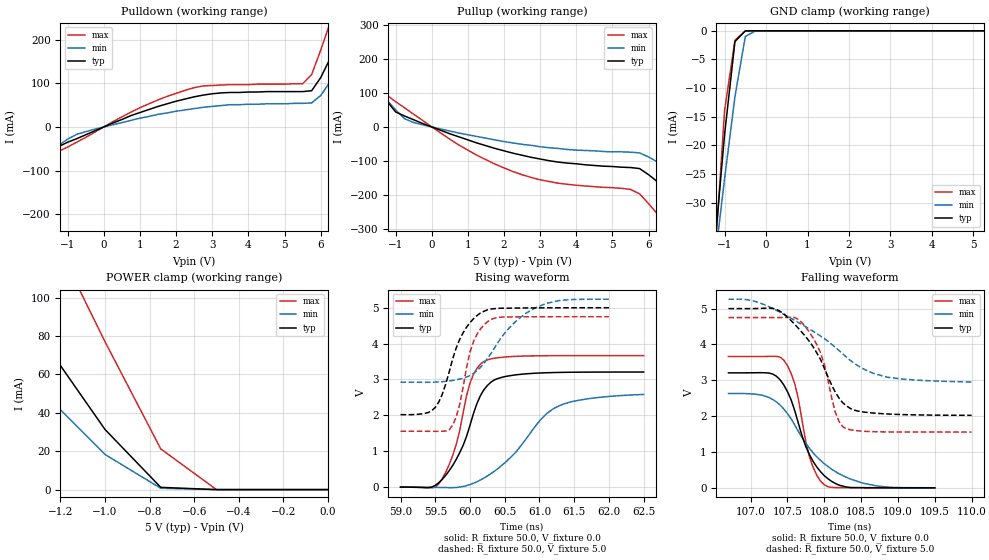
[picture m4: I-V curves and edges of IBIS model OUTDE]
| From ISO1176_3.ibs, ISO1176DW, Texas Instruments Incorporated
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[Model]   OUTDE
Model_type   3-state
| Signals   ISODE
Vmeas = 2.2V   |Reference voltage for timing measurements
Cref = 15pF   |Timing specification test load capacitance value
Vref = 0   |Timing specification test load voltage; GND
| variable   typ   min   max
C_comp   2.1pF   1.7pF   2.5pF
|   typ   min   max
[Temperature Range]   25.0   -40   125
[Voltage range]   5.0V   5.25V   4.75V
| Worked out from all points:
|   slope of the pulldown table from 0 to 0.75 V, typ, clamps not added: 28.8 ohm
|   slope of the pullup table from 0 to 0.75 V, typ, clamps not added: 25.9 ohm
|   GND clamp passes 1 mA (typ) near -0.63 V on its own axis
|   POWER clamp passes 1 mA (typ) near -0.71 V on its own axis
|   rising waveform, R_fixture 50.0, V_fixture 0.0: 20-80 % time 393ps typ, 714ps min, 285ps max; typ from 0.001 V to 3.21 V
|   falling waveform, R_fixture 50.0, V_fixture 0.0: 20-80 % time 354ps typ, 607ps min, 227ps max; typ from 3.21 V to 0 V
|   rising waveform, R_fixture 50.0, V_fixture 5.0: 20-80 % time 327ps typ, 586ps min, 227ps max; typ from 2.02 V to 5 V
|   falling waveform, R_fixture 50.0, V_fixture 5.0: 20-80 % time 497ps typ, 961ps min, 272ps max; typ from 5 V to 2.02 V
[Pulldown]
|   Voltage   I(typ)  I(min)  I(max)
-5.25V    -390mA     -298mA     -529mA
-4.25V    -301mA     -233mA     -406mA
-3.5V     -235mA     -185mA     -315mA
-2.75V    -169mA     -137mA     -223mA
-1.5V     -63mA      -58mA      -75mA
-750mV    -27mA      -17mA      -35mA
2.5V      69mA       42mA       90mA
5.5V      81mA       54mA       99mA
6.25V     155mA      102mA      236mA
6.75V     243mA      165mA      358mA
7.25V     333mA      231mA      483mA
10.5V     958mA      685mA      1.342A
[Pullup]
|   Voltage   I(typ)  I(min)  I(max)
| Note that the[Pullup]voltage table is referenced to Vcc
| and is calculated using Vtable=Vcc - Vmeasured.
-5.25V    791mA      609mA      1.061A
-3V       385mA      309mA      505mA
-2.5V     295mA      242mA      382mA
-2.25V    250mA      209mA      321mA
-1.25V    77mA       80mA       94mA
-1V       44mA       50mA       74mA
2.25V     -77mA      -47mA      -131mA
5.75V     -122mA     -76mA      -196mA
6.5V      -184mA     -119mA     -287mA
7.75V     -297mA     -201mA     -444mA
9.25V     -435mA     -301mA     -634mA
10.5V     -549mA     -384mA     -793mA
[GND_clamp]
|   Voltage   I(typ)   I(min)   I(max)
| Outputs in High Impedance (off)
-5.25V    -389mA     -298mA     -529mA
-1.25V    -38.6mA    -41.1mA    -41.5mA
-1V       -18.1mA    -25.8mA    -13.9mA
-750mV    -1.88mA    -11.5mA    -1.64mA
-500mV    -9.27uA    -986uA     -29.5uA
-250mV    -2.83nA    -1.59uA    -2.12nA
5.25V     59.6pA     2.04nA     374pA
[POWER_clamp]
|   Voltage  I(typ)   I(min)   I(max)
| Note that the [POWER_clamp] voltage table is referenced to Vcc
| and is calculated using Vtable = Vcc - Vmeasured.
| Outputs in Tri-state.
-5.25V    791mA      575mA      1.12A
-1.75V    160mA      111mA      258mA
-1.5V     116mA      78.7mA     197mA
-1.25V    72.9mA     47.4mA     136mA
-1V       31.3mA     18.3mA     77mA
-750mV    1.18mA     693uA      21.2mA
-500mV    96.1nA     841nA      9.4uA
0V        47.1pA     1.11nA     46.9pA
[Ramp]
|   typ   min   max
dV/dt_r   1.94V/0.39ns   1.59V/0.73ns   2.22V/0.28ns
dV/dt_f   1.94V/0.35ns   1.59V/0.61ns   2.22V/0.23ns
R_load = 50
[Rising Waveform]
R_fixture = 50.0
V_fixture = 0.0
C_fixture = 0p
L_fixture = 0n
|   V(typ)   V(min)   V(max)
59ns      627.5uV    504.9uV    -196.9nV
59.45ns   2.406mV    -5.873mV   -21.29mV
59.6ns    214.8mV    -10.74mV   231.2mV
59.8ns    766.5mV    -10.7mV    1.179V
60ns      1.726V     70.81mV    2.901V
60.2ns    2.712V     250.9mV    3.501V
60.45ns   3.055V     593.2mV    3.616V
61.2ns    3.193V     2.185V     3.663V
61.6ns    3.204V     2.433V     3.664V
62.5ns    3.208V     2.583V     3.664V
[Falling Waveform]
R_fixture = 50.0
V_fixture = 0.0
C_fixture = 0p
L_fixture = 0n
|   V(typ)   V(min)   V(max)
106.7ns   3.208V     2.632V     3.664V
107.2ns   3.202V     2.521V     3.667V
107.4ns   2.875V     2.202V     3.565V
107.6ns   2.154V     1.752V     2.905V
107.8ns   923.8mV    1.101V     864.5mV
107.9ns   580.2mV    862.2mV    348.9mV
108ns     340.1mV    675.1mV    87.48mV
108.2ns   76.21mV    395.3mV    6.018mV
108.6ns   5.4mV      121.1mV    572uV
109.5ns   224.2uV    3.3mV      -15.8uV
[Rising Waveform]
R_fixture = 50.0
V_fixture = 5.0
V_fixture_min = 5.25
V_fixture_max = 4.75
C_fixture = 0p
L_fixture = 0n
|   V(typ)   V(min)  V(max)
59ns      2.02V      2.926V     1.557V
59.45ns   2.132V     2.924V     1.555V
59.6ns    2.583V     2.939V     1.557V
59.7ns    3.206V     2.959V     1.598V
59.85ns   4.111V     3.01V      2.286V
60.05ns   4.693V     3.169V     4.054V
60.3ns    4.963V     3.72V      4.672V
60.6ns    4.989V     4.508V     4.744V
60.95ns   4.996V     5.006V     4.749V
62ns      5V         5.24V      4.75V
[Falling Waveform]
R_fixture = 50.0
V_fixture = 5.0
V_fixture_min = 5.25
V_fixture_max = 4.75
C_fixture = 0p
L_fixture = 0n
|   V(typ)   V(min)  V(max)
106.7ns   5V         5.259V     4.75V
107ns     5V         5.23V      4.75V
107.4ns   4.978V     4.954V     4.75V
107.7ns   4.332V     4.552V     4.602V
107.9ns   3.582V     4.234V     3.768V
108ns     3.342V     4.168V     3.462V
108.1ns   2.67V      3.921V     2.114V
108.3ns   2.29V      3.649V     1.646V
108.8ns   2.061V     3.088V     1.56V
110ns     2.023V     2.952V     1.556V
